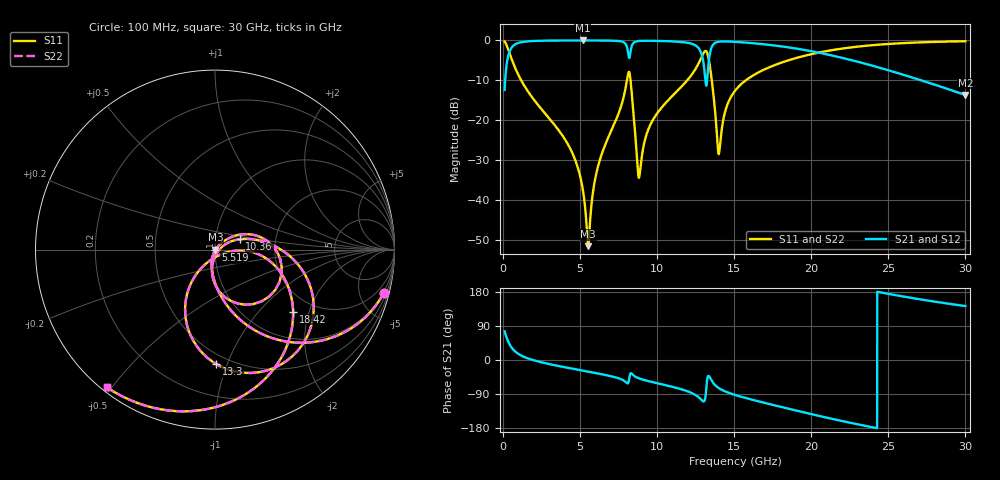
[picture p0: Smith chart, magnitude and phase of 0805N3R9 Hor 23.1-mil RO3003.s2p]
# GHz S MA R 50
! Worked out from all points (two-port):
!   3201 points, 100 MHz to 30 GHz, reference 50 ohm
!   highest |S21| = -0.02 dB at 5.155 GHz (marker M1); lowest = -13.7 dB at 30 GHz (marker M2)
!   |S21| within 3 dB of the highest: 401.5 MHz to 8.112 GHz (7.71 GHz wide, 181 % of centre); 13.44 GHz to 20.41 GHz (6.975 GHz wide, 41.2 % of centre)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
!   lowest |S11| = -51.5 dB at 5.529 GHz (marker M3), VSWR 1.01, Z = 50.2 - j0.126 ohm
!   |S11| at or under -10 dB: 1.175 GHz to 8.037 GHz (6.862 GHz wide, 149 % of centre); 8.272 GHz to 11.95 GHz (3.677 GHz wide, 36.4 % of centre); 13.54 GHz to 15.75 GHz (2.205 GHz wide, 15.1 % of centre)
!   |S22| runs from -51.5 to -0.2 dB; largest |S21 - S12| = 0
!   S11 on the Smith chart (normalised r, x): 100 MHz: 0.93, -7.76; 5.519 GHz: 1.00, -0.00; 10.36 GHz: 1.31, +0.15; 13.3 GHz: 0.43, -0.91; 18.42 GHz: 1.58, -1.58; 30 GHz: 0.02, -0.48
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0.1  0.9706 -14.5  0.2404 75.5  0.2404 75.5  0.9706 -14.5
0.4644063  0.6542 -51.7  0.7558 38.2  0.7558 38.2  0.6542 -51.7
1.183875  0.314 -78.2  0.9484 11.6  0.9484 11.6  0.314 -78.2
4.1365  0.05283 -107.9  0.9964 -20.1  0.9964 -20.1  0.05283 -107.9
5.089563  0.01677 -109.1  0.9973 -27.4  0.9973 -27.4  0.01677 -109.1
5.154969  0.01435 -108.0  0.9973 -27.9  0.9973 -27.9  0.01435 -108.0
5.519375  0.002665 -35.9  0.9971 -30.7  0.9971 -30.7  0.002665 -35.9
5.528719  0.002662 -28.2  0.9971 -30.7  0.9971 -30.7  0.002662 -28.2
6.15475  0.02622 47.4  0.9963 -35.6  0.9963 -35.6  0.02622 47.4
8.107594  0.3759 -11.4  0.7145 -61.1  0.7145 -61.1  0.3759 -11.4
8.827063  0.0192 -28.9  0.9816 -48.6  0.9816 -48.6  0.0192 -28.9
10.06978  0.1277 24.9  0.9843 -61.9  0.9843 -61.9  0.1277 24.9
10.35944  0.1498 22.7  0.9813 -64.6  0.9813 -64.6  0.1498 22.7
12.2095  0.3652 0.2  0.9102 -86.6  0.9102 -86.6  0.3652 0.2
12.89159  0.6221 -28.1  0.6626 -105.9  0.6626 -105.9  0.6221 -28.1
13.30272  0.6371 -89.5  0.4487 -42.8  0.4487 -42.8  0.6371 -89.5
14.0035  0.03788 -59.0  0.9629 -74.3  0.9629 -74.3  0.03788 -59.0
15.05  0.234 -5.4  0.9587 -92.2  0.9587 -92.2  0.234 -5.4
18.42309  0.5556 -38.5  0.8222 -127.6  0.8222 -127.6  0.5556 -38.5
20.03956  0.6742 -53.9  0.7291 -143.2  0.7291 -143.2  0.6742 -53.9
25.01978  0.9018 -96.2  0.4216 174.4  0.4216 174.4  0.9018 -96.2
30  0.9755 -128.3  0.2071 142.3  0.2071 142.3  0.9755 -128.3
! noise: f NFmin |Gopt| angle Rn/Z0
0.1  0.0008448  0.9279  1.227  0.0026
3.417  0.005964  0.6895  19.48  0.003634
6.743  0.01273  0.7148  37.07  0.007945
10.06  0.01993  0.7335  54.14  0.01191
13.39  0.1719  0.9551  70.88  0.5722
16.7  0.02945  0.7222  84.79  0.01171
20.03  0.03473  0.7284  97.97  0.01131
23.35  0.04487  0.7625  110.8  0.01284
26.67  0.06078  0.8073  123.5  0.01527
30  0.08685  0.8559  136.3  0.01849
